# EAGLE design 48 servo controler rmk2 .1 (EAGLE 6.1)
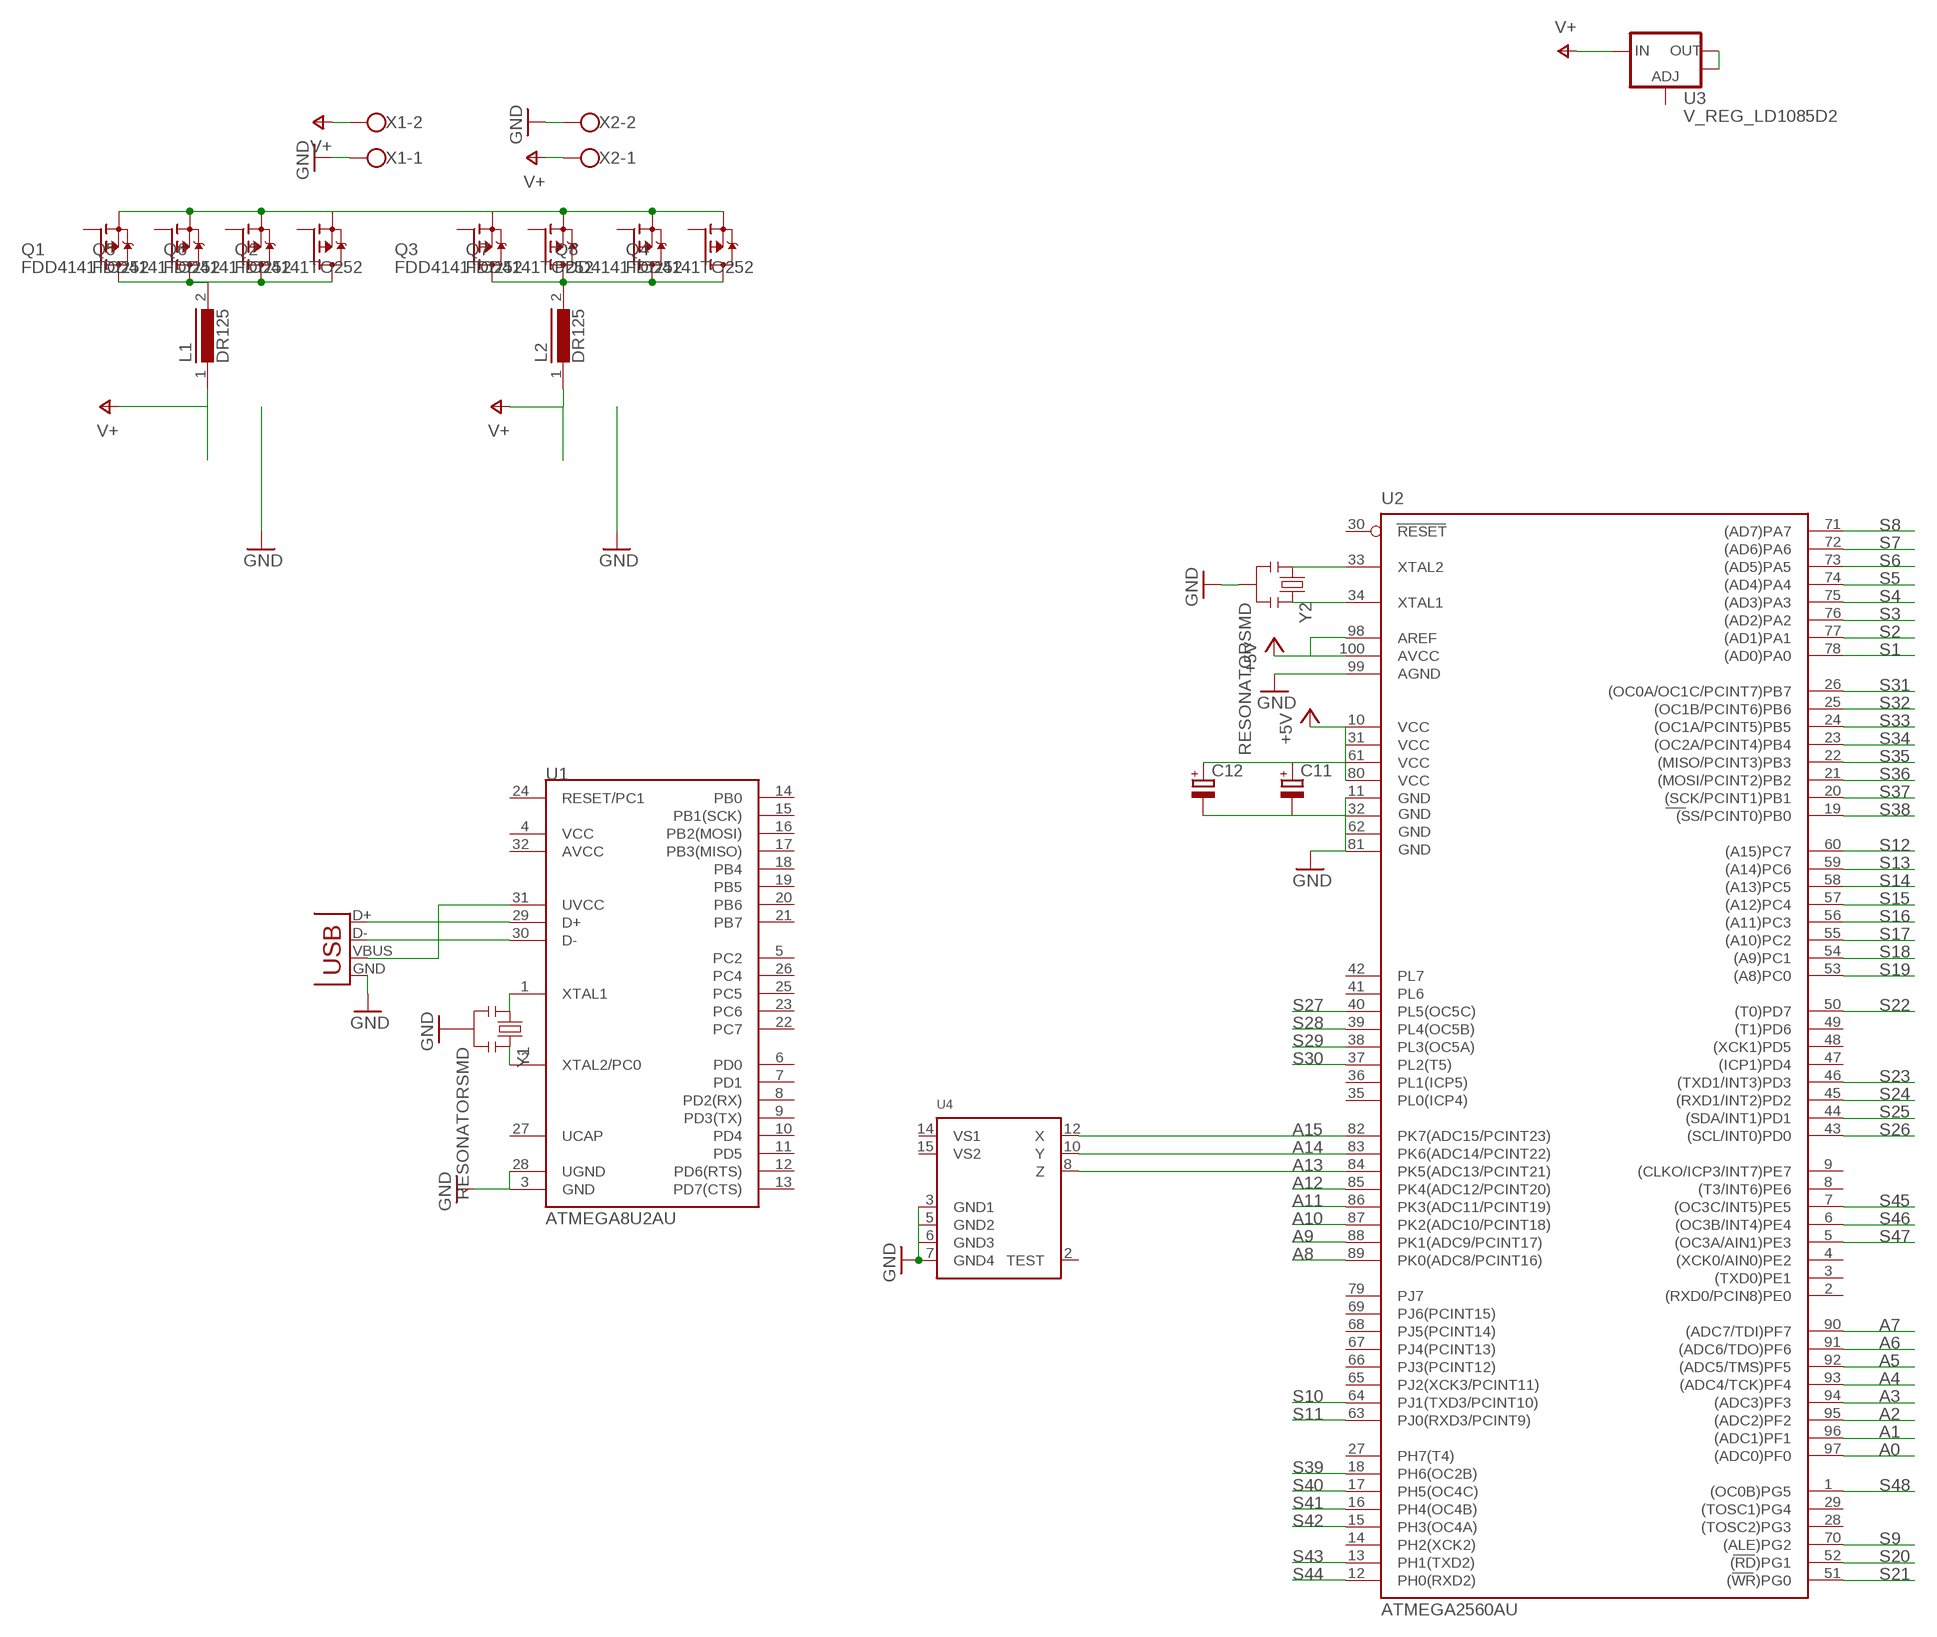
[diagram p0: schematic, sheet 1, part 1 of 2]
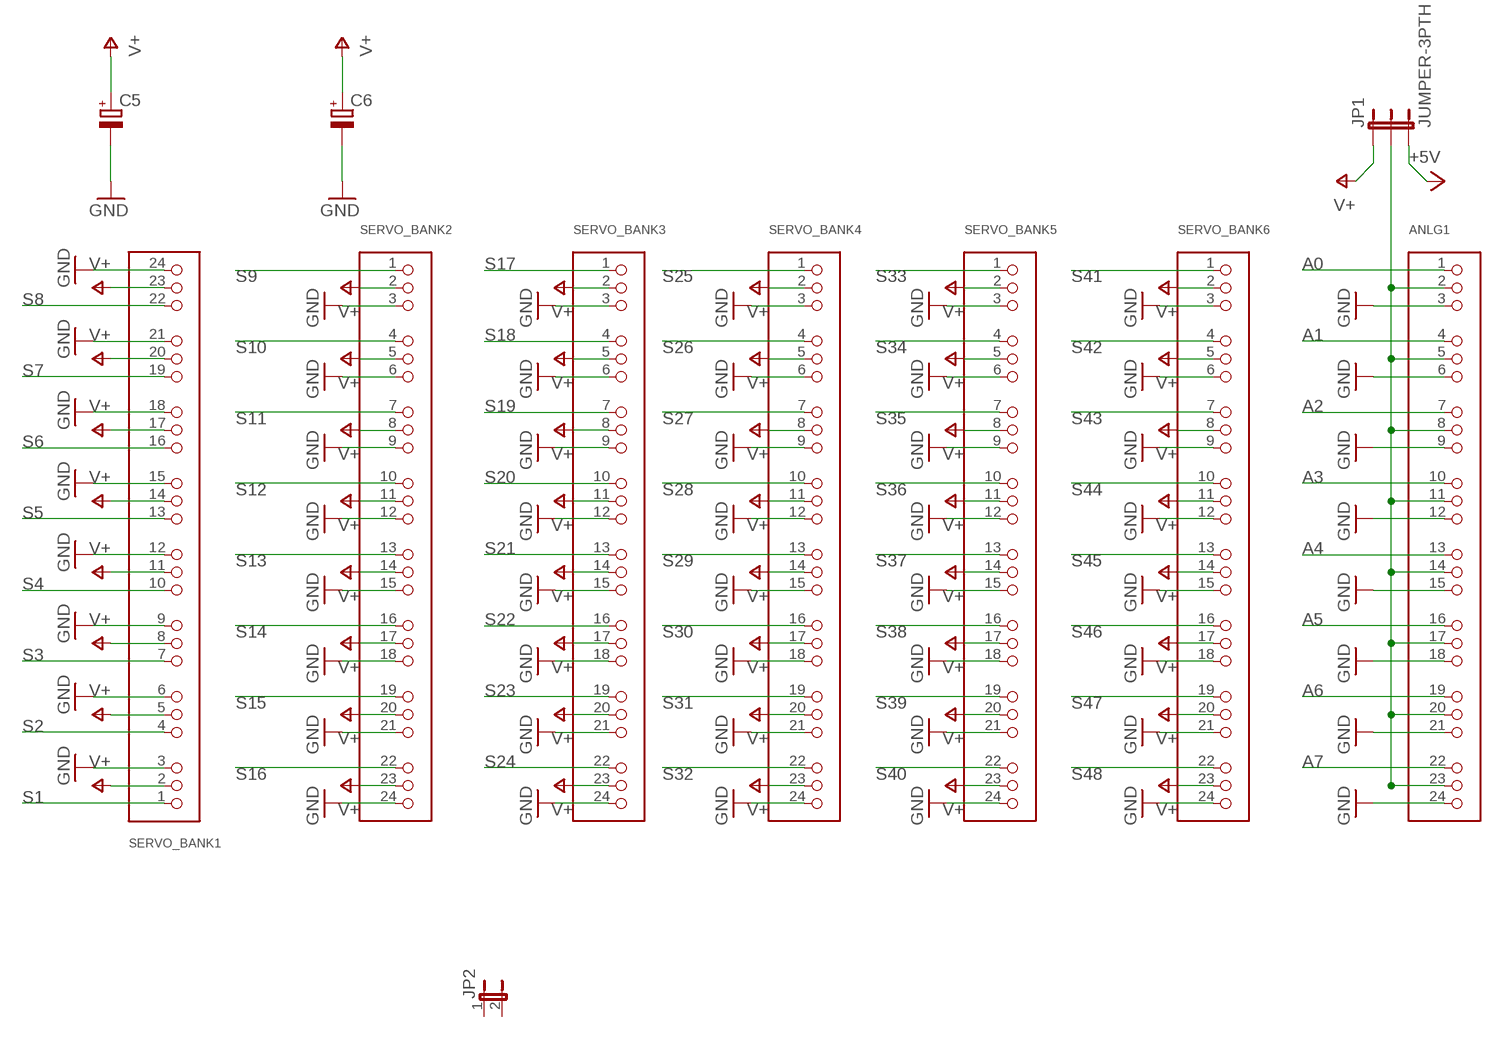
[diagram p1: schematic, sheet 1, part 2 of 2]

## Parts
ANLG1  HEADER-3X08  [3X08]
C5  CPOL-EUE5-8.5  [E5-8,5]
C6  CPOL-EUE5-8.5  [E5-8,5]
C11  CPOL-EUSMCE  [SMC_E]
C12  CPOL-EUSMCE  [SMC_E]
JP1  JUMPER-3PTH  [1X03]
JP2  JP1E  [JP1]
L1  DR125  [DR125]
L2  DR125  [DR125]
Q1  FDD4141TO252  [TO252]
Q2  FDD4141TO252  [TO252]
Q3  FDD4141TO252  [TO252]
Q4  FDD4141TO252  [TO252]
Q5  FDD4141TO252  [TO252]
Q6  FDD4141TO252  [TO252]
Q7  FDD4141TO252  [TO252]
Q8  FDD4141TO252  [TO252]
SERVO_BANK1  HEADER-3X08  [3X08]
SERVO_BANK2  HEADER-3X08  [3X08]
SERVO_BANK3  HEADER-3X08  [3X08]
SERVO_BANK4  HEADER-3X08  [3X08]
SERVO_BANK5  HEADER-3X08  [3X08]
SERVO_BANK6  HEADER-3X08  [3X08]
U1  ATMEGA8U2AU  [TQFP32-08]
U2  ATMEGA2560AU  [TQFP100]
U3  V_REG_LD1085D2  [D2PACK/A]
U4  ACCEL_ADXL335WAVE  [LFCSP16-W]
X1  W237-102  [W237-102]
X2  W237-102  [W237-102]
X4  USBSMD  [USB-MINIB]
Y1  RESONATORSMD  [RESONATOR-SMD]
Y2  RESONATORSMD  [RESONATOR-SMD]

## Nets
+5V: C11.+ C12.+ JP1.3 U2.10(VCC) U2.31(VCC1) U2.61(VCC2) U2.80(VCC3) U2.98(AREF) U2.100(AVCC)
A0: ANLG1.1 U2.97((ADC0)PF0)
A1: ANLG1.4 U2.96((ADC1)PF1)
A2: ANLG1.7 U2.95((ADC2)PF2)
A3: ANLG1.10 U2.94((ADC3)PF3)
A4: ANLG1.13 U2.93((ADC4/TCK)PF4)
A5: ANLG1.16 U2.92((ADC5/TMS)PF5)
A6: ANLG1.19 U2.91((ADC6/TDO)PF6)
A7: ANLG1.22 U2.90((ADC7/TDI)PF7)
A8: U2.89(PK0(ADC8/PCINT16))
A9: U2.88(PK1(ADC9/PCINT17))
A10: U2.87(PK2(ADC10/PCINT18))
A11: U2.86(PK3(ADC11/PCINT19))
A12: U2.85(PK4(ADC12/PCINT20))
A13: U2.84(PK5(ADC13/PCINT21)) U4.8(Z)
A14: U2.83(PK6(ADC14/PCINT22)) U4.10(Y)
A15: U2.82(PK7(ADC15/PCINT23)) U4.12(X)
GND: ANLG1.3 ANLG1.6 ANLG1.9 ANLG1.12 ANLG1.15 ANLG1.18 ANLG1.21 ANLG1.24 C5.- C6.- C11.- C12.- SERVO_BANK1.3 SERVO_BANK1.6 SERVO_BANK1.9 SERVO_BANK1.12 SERVO_BANK1.15 SERVO_BANK1.18 SERVO_BANK1.21 SERVO_BANK1.24 SERVO_BANK2.3 SERVO_BANK2.6 SERVO_BANK2.9 SERVO_BANK2.12 SERVO_BANK2.15 SERVO_BANK2.18 SERVO_BANK2.21 SERVO_BANK2.24 SERVO_BANK3.3 SERVO_BANK3.6 SERVO_BANK3.9 SERVO_BANK3.12 SERVO_BANK3.15 SERVO_BANK3.18 SERVO_BANK3.21 SERVO_BANK3.24 SERVO_BANK4.3 SERVO_BANK4.6 SERVO_BANK4.9 SERVO_BANK4.12 SERVO_BANK4.15 SERVO_BANK4.18 SERVO_BANK4.21 SERVO_BANK4.24 SERVO_BANK5.3 SERVO_BANK5.6 SERVO_BANK5.9 SERVO_BANK5.12 SERVO_BANK5.15 SERVO_BANK5.18 SERVO_BANK5.21 SERVO_BANK5.24 SERVO_BANK6.3 SERVO_BANK6.6 SERVO_BANK6.9 SERVO_BANK6.12 SERVO_BANK6.15 SERVO_BANK6.18 SERVO_BANK6.21 SERVO_BANK6.24 U1.3(GND) U1.28(UGND) U2.11(GND) U2.32(GND1) U2.62(GND2) U2.81(GND3) U2.99(AGND) U4.3(GND1) U4.5(GND2) U4.6(GND3) U4.7(GND4) X1.1 X2.2 X4.GND Y1.2 Y2.2
N$1: U2.34(XTAL1) Y2.3
N$2: U2.33(XTAL2) Y2.1
N$3: U1.2(XTAL2/PC0) Y1.3
N$4: U1.1(XTAL1) Y1.1
N$5: U3.2(OUT) U3.TAB(OUT)
N$9: U1.29(D+) X4.D+
N$10: ANLG1.2 ANLG1.5 ANLG1.8 ANLG1.11 ANLG1.14 ANLG1.17 ANLG1.20 ANLG1.23 JP1.2
N$11: U1.30(D-) X4.D-
N$12: U1.31(UVCC) X4.VBUS
N$49: L2.2 Q3.3(D) Q4.3(D) Q7.3(D) Q8.3(D)
N$50: L1.2 Q1.3(D) Q2.3(D) Q5.3(D) Q6.3(D)
N$51: Q1.2(S) Q2.2(S) Q3.2(S) Q4.2(S) Q5.2(S) Q6.2(S) Q7.2(S) Q8.2(S)
S1: SERVO_BANK1.1 U2.78((AD0)PA0)
S2: SERVO_BANK1.4 U2.77((AD1)PA1)
S3: SERVO_BANK1.7 U2.76((AD2)PA2)
S4: SERVO_BANK1.10 U2.75((AD3)PA3)
S5: SERVO_BANK1.13 U2.74((AD4)PA4)
S6: SERVO_BANK1.16 U2.73((AD5)PA5)
S7: SERVO_BANK1.19 U2.72((AD6)PA6)
S8: SERVO_BANK1.22 U2.71((AD7)PA7)
S9: SERVO_BANK2.1 U2.70((ALE)PG2)
S10: SERVO_BANK2.4 U2.64(PJ1(TXD3/PCINT10))
S11: SERVO_BANK2.7 U2.63(PJ0(RXD3/PCINT9))
S12: SERVO_BANK2.10 U2.60((A15)PC7)
S13: SERVO_BANK2.13 U2.59((A14)PC6)
S14: SERVO_BANK2.16 U2.58((A13)PC5)
S15: SERVO_BANK2.19 U2.57((A12)PC4)
S16: SERVO_BANK2.22 U2.56((A11)PC3)
S17: SERVO_BANK3.1 U2.55((A10)PC2)
S18: SERVO_BANK3.4 U2.54((A9)PC1)
S19: SERVO_BANK3.7 U2.53((A8)PC0)
S20: SERVO_BANK3.10 U2.52((RD)PG1)
S21: SERVO_BANK3.13 U2.51((WR)PG0)
S22: SERVO_BANK3.16 U2.50((T0)PD7)
S23: SERVO_BANK3.19 U2.46((TXD1/INT3)PD3)
S24: SERVO_BANK3.22 U2.45((RXD1/INT2)PD2)
S25: SERVO_BANK4.1 U2.44((SDA/INT1)PD1)
S26: SERVO_BANK4.4 U2.43((SCL/INT0)PD0)
S27: SERVO_BANK4.7 U2.40(PL5(OC5C))
S28: SERVO_BANK4.10 U2.39(PL4(OC5B))
S29: SERVO_BANK4.13 U2.38(PL3(OC5A))
S30: SERVO_BANK4.16 U2.37(PL2(T5))
S31: SERVO_BANK4.19 U2.26((OC0A/OC1C/PCINT7)PB7)
S32: SERVO_BANK4.22 U2.25((OC1B/PCINT6)PB6)
S33: SERVO_BANK5.1 U2.24((OC1A/PCINT5)PB5)
S34: SERVO_BANK5.4 U2.23((OC2A/PCINT4)PB4)
S35: SERVO_BANK5.7 U2.22((MISO/PCINT3)PB3)
S36: SERVO_BANK5.10 U2.21((MOSI/PCINT2)PB2)
S37: SERVO_BANK5.13 U2.20((SCK/PCINT1)PB1)
S38: SERVO_BANK5.16 U2.19((SS/PCINT0)PB0)
S39: SERVO_BANK5.19 U2.18(PH6(OC2B))
S40: SERVO_BANK5.22 U2.17(PH5(OC4C))
S41: SERVO_BANK6.1 U2.16(PH4(OC4B))
S42: SERVO_BANK6.4 U2.15(PH3(OC4A))
S43: SERVO_BANK6.7 U2.13(PH1(TXD2))
S44: SERVO_BANK6.10 U2.12(PH0(RXD2))
S45: SERVO_BANK6.13 U2.7((OC3C/INT5)PE5)
S46: SERVO_BANK6.16 U2.6((OC3B/INT4)PE4)
S47: SERVO_BANK6.19 U2.5((OC3A/AIN1)PE3)
S48: SERVO_BANK6.22 U2.1((OC0B)PG5)
V+: C5.+ C6.+ JP1.1 L1.1 L2.1 SERVO_BANK1.2 SERVO_BANK1.5 SERVO_BANK1.8 SERVO_BANK1.11 SERVO_BANK1.14 SERVO_BANK1.17 SERVO_BANK1.20 SERVO_BANK1.23 SERVO_BANK2.2 SERVO_BANK2.5 SERVO_BANK2.8 SERVO_BANK2.11 SERVO_BANK2.14 SERVO_BANK2.17 SERVO_BANK2.20 SERVO_BANK2.23 SERVO_BANK3.2 SERVO_BANK3.5 SERVO_BANK3.8 SERVO_BANK3.11 SERVO_BANK3.14 SERVO_BANK3.17 SERVO_BANK3.20 SERVO_BANK3.23 SERVO_BANK4.2 SERVO_BANK4.5 SERVO_BANK4.8 SERVO_BANK4.11 SERVO_BANK4.14 SERVO_BANK4.17 SERVO_BANK4.20 SERVO_BANK4.23 SERVO_BANK5.2 SERVO_BANK5.5 SERVO_BANK5.8 SERVO_BANK5.11 SERVO_BANK5.14 SERVO_BANK5.17 SERVO_BANK5.20 SERVO_BANK5.23 SERVO_BANK6.2 SERVO_BANK6.5 SERVO_BANK6.8 SERVO_BANK6.11 SERVO_BANK6.14 SERVO_BANK6.17 SERVO_BANK6.20 SERVO_BANK6.23 U3.3(IN) X1.2 X2.1
Unconnected: JP2.1 JP2.2 Q1.1(G) Q2.1(G) Q3.1(G) Q4.1(G) Q5.1(G) Q6.1(G) Q7.1(G) Q8.1(G) U1.4(VCC) U1.5(PC2) U1.6(PD0) U1.7(PD1) U1.8(PD2(RX)) U1.9(PD3(TX)) U1.10(PD4) U1.11(PD5) U1.12(PD6(RTS)) U1.13(PD7(CTS)) U1.14(PB0) U1.15(PB1(SCK)) U1.16(PB2(MOSI)) U1.17(PB3(MISO)) U1.18(PB4) U1.19(PB5) U1.20(PB6) U1.21(PB7) U1.22(PC7) U1.23(PC6) U1.24(RESET/PC1) U1.25(PC5) U1.26(PC4) U1.27(UCAP) U1.32(AVCC) U2.2((RXD0/PCIN8)PE0) U2.3((TXD0)PE1) U2.4((XCK0/AIN0)PE2) U2.8((T3/INT6)PE6) U2.9((CLKO/ICP3/INT7)PE7) U2.14(PH2(XCK2)) U2.27(PH7(T4)) U2.28((TOSC2)PG3) U2.29((TOSC1)PG4) U2.30(RESET) U2.35(PL0(ICP4)) U2.36(PL1(ICP5)) U2.41(PL6) U2.42(PL7) U2.47((ICP1)PD4) U2.48((XCK1)PD5) U2.49((T1)PD6) U2.65(PJ2(XCK3/PCINT11)) U2.66(PJ3(PCINT12)) U2.67(PJ4(PCINT13)) U2.68(PJ5(PCINT14)) U2.69(PJ6(PCINT15)) U2.79(PJ7) U3.1(ADJ) U4.2(TEST) U4.14(VS1) U4.15(VS2)

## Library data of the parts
ANLG1 SERVO_BANK1-SERVO_BANK6 = microbuilder:HEADER-3X08: 3x8 0.1" Headers Male - 4UCON: 01058
C5 C6 C11 C12 = resistor:CPOL-EU: POLARIZED CAPACITOR, European symbol
JP1 = SparkFun:JUMPER-3
JP2 = jumper:JP1E: JUMPER
L1 L2 = inductors:DR125: High Power Density, High Efficiency, Shielded Inductors
Q1-Q8 = transistor-fet:FDD4141: P-Channel PowerTrench® MOSFET Source: FDD4141.pdf
U1 = SparkFun:ATMEGA8U2: Atmel 8-bit Microcontroller with 8/16/32K Bystes of ISP Flash and USB Controller. ATmega8U2, ATmega16U2, and ATmega32U2
U2 = SparkFun:ATMEGA2560: MICROCONTROLLER 64/128/256 Kbytes FLASH 4 Kbytes EEPROM 8 Kbytes SRAM 86 General Purpose I/O pins 12-channels16-bit PWM 4 x Serial USARTs 16-channels 10-bit A/D
U3 = SparkFun:V_REG_LD1085: LD1085 3A low-drop positive voltage regulator, adjustable The LD1085xx is a low drop voltage regulator able to provide up to 3 A of output current. Dropout is guaranteed at a maximum of 1.2 V at the maximum output current, decreasing at lower loads. The LD1085xx is pin to pin compatible with the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
U4 = microbuilder:ACCEL_ADXL335: ADXL335 Low-Power 3 Axis Accelerometer LFCSP16-R - 16 Pin LFCSP Package (Reflow footprint) LFSCP16-W - 16 Pin LFCSP Package (Wave footprint with extended pads for hand soldering) Digikey: ADXL335BCPZ-RL7CT-ND
X1 X2 = con-wago-500:W237-102: WAGO SCREW CLAMP; MPN: 237-102; OC_FARNELL: unknown; OC_NEWARK: 70K9898
X4 = SparkFun:USB: USB Connectors USB-B-PTH is fully proven SKU : PRT-00139 USB-miniB is fully proven SKU : PRT-00587 USB-A-PCB is untested. USB-A-H is throughly reviewed, but untested. Spark Fun Electronics SKU : PRT-00437 USB-B-SMT is throughly reviewed, but untested. Needs silkscreen touching up. USB-A-S has not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
Y1 Y2 = SparkFun:RESONATOR: Resonator Small SMD resonator. This is the itty bitty 10/20MHz resonators with built in caps. CSTCE10M0G55 and CSTCE20M0V53. Footprint has been reviewed closely but hasn't been tested yet.

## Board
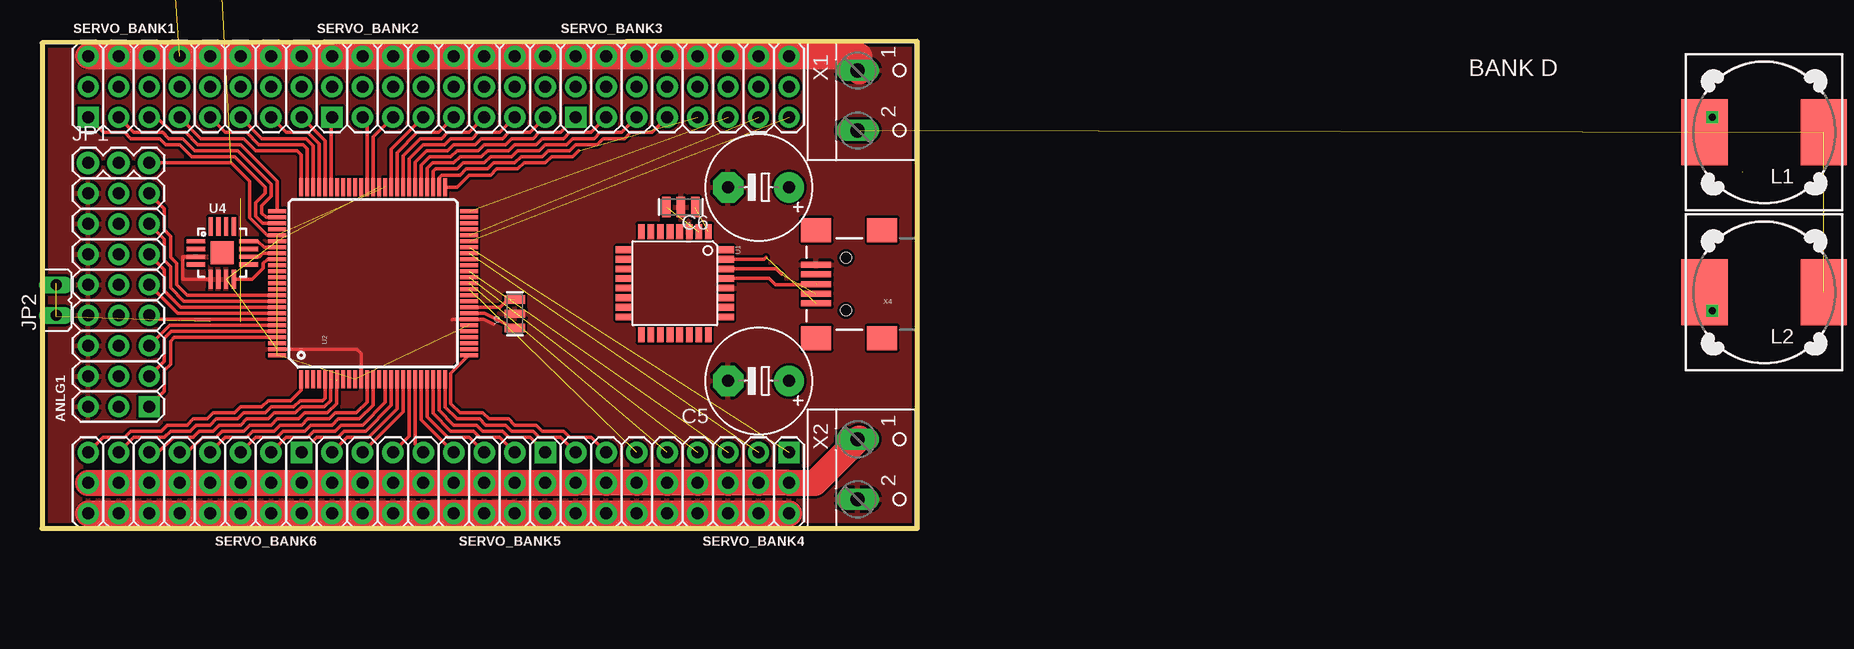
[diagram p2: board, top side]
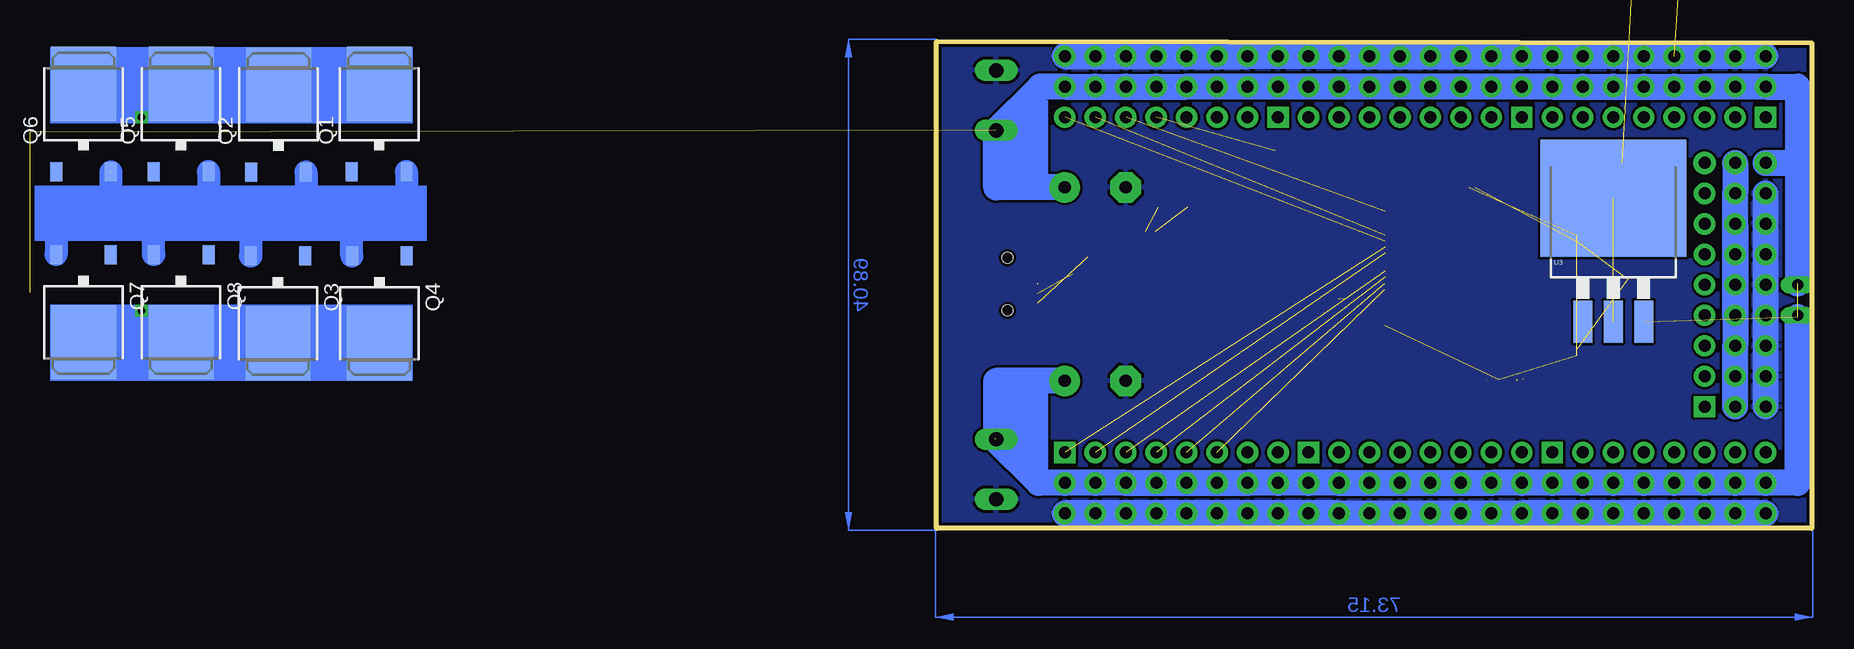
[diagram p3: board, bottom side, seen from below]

Size 72.95 x 40.57 mm. Coordinates in mm from the lower left corner, seen from the top.
Outline: 0,40.44 0,0 72.95,0 72.95,40.57 0,40.44
Copper layers (1*16): Top 0.035mm / dielectric 1.5mm / Bottom 0.035mm
Design rules: minimum track width 10mil, minimum drill 24mil, track to track 8mil, track to pad 8mil, pad to pad 8mil, via to via 8mil, smd to smd 8mil, copper to edge 10mil, drill to drill 8mil, minimum pad ring 10mil, minimum via ring 8mil, stop-mask expansion 4mil, vias tented up to drill 0mil, thermal gap 10mil

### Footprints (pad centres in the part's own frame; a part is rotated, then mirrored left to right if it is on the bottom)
3X08 = drill 1 pad 1.778 square: 1 -8.89,-2.54 | drill 1 pad 1.778: 2 -8.89,0; 3 -8.89,2.54; 4 -6.35,-2.54; 5 -6.35,0; 6 -6.35,2.54; 7 -3.81,-2.54; 8 -3.81,0; 9 -3.81,2.54; 10 -1.27,-2.54; 11 -1.27,0; 12 -1.27,2.54; 13 1.27,-2.54; 14 1.27,0; 15 1.27,2.54; 16 3.81,-2.54; 17 3.81,0; 18 3.81,2.54; 19 6.35,-2.54; 20 6.35,0; 21 6.35,2.54; 22 8.89,-2.54; 23 8.89,0; 24 8.89,2.54
E5-8,5 = drill 1.016 pad 2.54: + -2.54,0 | drill 1.016 pad 2.54 octagon: - 2.54,0
SMC_E = smd 2.4 x 2.8: + -3.15,0; - 3.15,0
1X03 = drill 1.016 pad 1.88: 1 0,0; 2 2.54,0; 3 5.08,0
JP1 = drill 0.914 long: 1 0,-1.27; 2 0,1.27
DR125 = smd 3.85 x 5.5: 1 -4.975,0; 2 4.975,0
TO252 = smd 1 x 1.6: 1 -2.28,-4.8; 2 2.28,-4.8 | smd 5.4 x 6.2: 3 0,2.5
TQFP32-08 = smd 1.27 x 0.559: 1 -4.293,2.8; 2 -4.293,2; 3 -4.293,1.2; 4 -4.293,0.4; 5 -4.293,-0.4; 6 -4.293,-1.2; 7 -4.293,-2; 8 -4.293,-2.8; 17 4.293,-2.8; 18 4.293,-2; 19 4.293,-1.2; 20 4.293,-0.4; 21 4.293,0.4; 22 4.293,1.2; 23 4.293,2; 24 4.293,2.8 | smd 0.559 x 1.27: 9 -2.8,-4.293; 10 -2,-4.293; 11 -1.2,-4.293; 12 -0.4,-4.293; 13 0.4,-4.293; 14 1.2,-4.293; 15 2,-4.293; 16 2.8,-4.293; 25 2.8,4.293; 26 2,4.293; 27 1.2,4.293; 28 0.4,4.293; 29 -0.4,4.293; 30 -1.2,4.293; 31 -2,4.293; 32 -2.8,4.293
TQFP100 = smd 1.5 x 0.3: 1 -8,6; 2 -8,5.5; 3 -8,5; 4 -8,4.5; 5 -8,4; 6 -8,3.5; 7 -8,3; 8 -8,2.5; 9 -8,2; 10 -8,1.5; 11 -8,1; 12 -8,0.5; 13 -8,0; 14 -8,-0.5; 15 -8,-1; 16 -8,-1.5; 17 -8,-2; 18 -8,-2.5; 19 -8,-3; 20 -8,-3.5; 21 -8,-4; 22 -8,-4.5; 23 -8,-5; 24 -8,-5.5; 25 -8,-6; 51 8,-6; 52 8,-5.5; 53 8,-5; 54 8,-4.5; 55 8,-4; 56 8,-3.5; 57 8,-3; 58 8,-2.5; 59 8,-2; 60 8,-1.5; 61 8,-1; 62 8,-0.5; 63 8,0; 64 8,0.5; 65 8,1; 66 8,1.5; 67 8,2; 68 8,2.5; 69 8,3; 70 8,3.5; 71 8,4; 72 8,4.5; 73 8,5; 74 8,5.5; 75 8,6 | smd 0.3 x 1.5: 26 -6,-8; 27 -5.5,-8; 28 -5,-8; 29 -4.5,-8; 30 -4,-8; 31 -3.5,-8; 32 -3,-8; 33 -2.5,-8; 34 -2,-8; 35 -1.5,-8; 36 -1,-8; 37 -0.5,-8; 38 0,-8; 39 0.5,-8; 40 1,-8; 41 1.5,-8; 42 2,-8; 43 2.5,-8; 44 3,-8; 45 3.5,-8; 46 4,-8; 47 4.5,-8; 48 5,-8; 49 5.5,-8; 50 6,-8; 76 6,8; 77 5.5,8; 78 5,8; 79 4.5,8; 80 4,8; 81 3.5,8; 82 3,8; 83 2.5,8; 84 2,8; 85 1.5,8; 86 1,8; 87 0.5,8; 88 0,8; 89 -0.5,8; 90 -1,8; 91 -1.5,8; 92 -2,8; 93 -2.5,8; 94 -3,8; 95 -3.5,8; 96 -4,8; 97 -4.5,8; 98 -5,8; 99 -5.5,8; 100 -6,8
D2PACK/A = smd 1.6 x 3.5: 1 -2.54,-8.275; 2 0,-8.275; 3 2.54,-8.275 | smd 12.2 x 9.75: TAB 0,2
LFCSP16-W = smd 1.9 x 1.9: 0 0,0 | smd 1.558 x 0.35: 1 -2.204,0.975; 2 -2.204,0.325; 3 -2.204,-0.325; 4 -2.204,-0.975; 9 2.204,-0.975; 10 2.204,-0.325; 11 2.204,0.325; 12 2.204,0.975 | smd 0.35 x 1.558: 5 -0.975,-2.204; 6 -0.325,-2.204; 7 0.325,-2.204; 8 0.975,-2.204; 13 0.975,2.204; 14 0.325,2.204; 15 -0.325,2.204; 16 -0.975,2.204
W237-102 = drill 1.194 long: 1 -2.5,-1.27; 2 2.5,-1.27
USB-MINIB = smd 2.5 x 0.5: D+ 2.5,0; D- 2.5,0.8; GND 2.5,-1.6; ID 2.5,-0.8; VBUS 2.5,1.6 | smd 2.5 x 2: MTN1 -3,4.5; MTN2 2.5,4.5; MTN3 -3,-4.5; MTN4 2.5,-4.5 | hole 0.9: 0,2.2; 0,-2.2
RESONATOR-SMD = smd 0.7 x 1.7: 1 -1.2,0; 2 0,0; 3 1.2,0

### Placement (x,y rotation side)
ANLG1  6.38,19.02 90 top
C5  59.72,12.29 180 top
C6  59.72,28.42 180 top
C11  not placed on the board
C12  not placed on the board
JP1  3.84,30.45 0 top
JP2  1.17,19.02 0 top
L1  143.54,32.99 180 top  (outside the outline)
L2  143.54,19.65 180 top  (outside the outline)
Q1  119.41,34.51 0 bottom  (outside the outline)
Q2  127.79,34.48 0 bottom  (outside the outline)
Q3  127.85,17.91 180 bottom  (outside the outline)
Q4  119.4,17.91 180 bottom  (outside the outline)
Q5  135.92,34.51 0 bottom  (outside the outline)
Q6  144.05,34.51 0 bottom  (outside the outline)
Q7  144.05,18 180 bottom  (outside the outline)
Q8  135.92,18 180 bottom  (outside the outline)
SERVO_BANK1  12.73,36.8 0 top
SERVO_BANK2  33.05,36.8 0 top
SERVO_BANK3  53.37,36.8 0 top
SERVO_BANK4  53.37,3.78 180 top
SERVO_BANK5  33.05,3.78 180 top
SERVO_BANK6  12.73,3.78 180 top
U1  52.73,20.41 270 top
U2  27.59,20.41 90 top
U3  16.54,25.49 0 bottom
U4  15.01,22.95 0 top
X1  69.24,35.65 270 top
X2  69.24,4.92 270 top
X4  67.02,20.35 180 top
Y1  53.24,26.76 180 top
Y2  39.4,17.87 90 top

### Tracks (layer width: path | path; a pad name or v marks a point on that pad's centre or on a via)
+5V  (7 unrouted)
  Top 0.305: U2.80 18.76,24.41 17.3,25.88 17.3,28.92 15.78,30.45 JP1.3
A0
  Top 0.305: U2.97 11.02,15.91 10.7,15.59 10.7,13.68 10.19,13.17 10.19,11.4 ANLG1.1
A1
  Top 0.305: U2.96 10.76,16.41 10.19,15.84 10.19,13.94 ANLG1.4
A2
  Top 0.305: U2.95 10.62,16.91 ANLG1.7
A3
  Top 0.305: U2.94 9.25,17.41 ANLG1.10
A4
  Top 0.305: U2.93 11.29,17.91 ANLG1.13
A5
  Top 0.305: U2.92 11.55,18.41 10.19,19.78 10.19,21.56 ANLG1.16
A6
  Top 0.305: U2.91 11.81,18.91 10.7,20.03 10.7,21.81 10.19,22.32 10.19,24.1 ANLG1.19
A7
  Top 0.305: U2.90 12.08,19.41 11.2,20.29 11.2,22.07 10.7,22.57 10.7,24.35 10.19,24.86 10.19,26.64 ANLG1.22
A13
  Top 0.305: U4.8 17.51,20.75 18.44,21.68 18.44,22.07 18.79,22.41 U2.84
A14
  Top 0.305: U4.10 18.12,22.63 18.4,22.91 U2.83
A15
  Top 0.305: U2.82 18.49,23.41 17.98,23.93 U4.12
GND  (5 unrouted)
  Top 0.305: 37.62,16.98 36.81,17.41 U2.32 34.24,17.41 34.19,17.37 | U2.99 26.23,14.91 26.57,14.57 26.57,12.43 U2.11 | U4.3 11.71,22.63 11.71,20.75 U4.5
  Top 2.184: SERVO_BANK6.24 SERVO_BANK6.21 SERVO_BANK6.18 SERVO_BANK6.15 SERVO_BANK6.12 SERVO_BANK6.9 SERVO_BANK6.6 SERVO_BANK6.3 SERVO_BANK5.24 SERVO_BANK5.21 SERVO_BANK5.18 SERVO_BANK5.15 SERVO_BANK5.12 SERVO_BANK5.9 SERVO_BANK5.6 SERVO_BANK5.3 SERVO_BANK4.24 SERVO_BANK4.21 SERVO_BANK4.18 SERVO_BANK4.15 SERVO_BANK4.12 SERVO_BANK4.9 SERVO_BANK4.6 SERVO_BANK4.3 | SERVO_BANK1.3 SERVO_BANK1.6 SERVO_BANK1.9 SERVO_BANK1.12 SERVO_BANK1.15 SERVO_BANK1.18 SERVO_BANK1.21 SERVO_BANK1.24 SERVO_BANK2.3 SERVO_BANK2.6 SERVO_BANK2.9 SERVO_BANK2.12 SERVO_BANK2.15 SERVO_BANK2.18 SERVO_BANK2.21 SERVO_BANK2.24 SERVO_BANK3.3 SERVO_BANK3.6 SERVO_BANK3.9 SERVO_BANK3.12 SERVO_BANK3.15 SERVO_BANK3.18 SERVO_BANK3.21 SERVO_BANK3.24 68.1,39.34 68.1,38.07
  Bottom 2.184: SERVO_BANK1.3 SERVO_BANK1.6 SERVO_BANK1.9 SERVO_BANK1.12 SERVO_BANK1.15 SERVO_BANK1.18 SERVO_BANK1.21 SERVO_BANK1.24 SERVO_BANK2.3 SERVO_BANK2.6 SERVO_BANK2.9 SERVO_BANK2.12 SERVO_BANK2.15 SERVO_BANK2.18 SERVO_BANK2.21 SERVO_BANK2.24 SERVO_BANK3.3 SERVO_BANK3.6 SERVO_BANK3.9 SERVO_BANK3.12 SERVO_BANK3.15 SERVO_BANK3.18 SERVO_BANK3.21 SERVO_BANK3.24 | SERVO_BANK4.24 SERVO_BANK4.21 SERVO_BANK4.18 SERVO_BANK4.15 | SERVO_BANK4.15 SERVO_BANK4.12 SERVO_BANK4.9 SERVO_BANK4.6 SERVO_BANK4.3 | SERVO_BANK4.24 SERVO_BANK4.15 | SERVO_BANK6.24 SERVO_BANK6.21 SERVO_BANK6.18 SERVO_BANK6.15 SERVO_BANK6.12 SERVO_BANK6.9 SERVO_BANK6.6 SERVO_BANK6.3 SERVO_BANK5.24 SERVO_BANK5.21 SERVO_BANK5.18 SERVO_BANK5.15 SERVO_BANK5.12 SERVO_BANK5.9 SERVO_BANK5.6 SERVO_BANK5.3 SERVO_BANK4.24 | ANLG1.3 ANLG1.6 ANLG1.9 ANLG1.12 ANLG1.15 ANLG1.18 ANLG1.21 ANLG1.24
  pour Top: -0.1,40.48 73.05,40.73 73.05,-0.16 -0.1,-0.16
  pour Bottom: 0.15,40.35 72.93,40.35 72.93,0.09 0.28,0.09 0.28,40.23
N$1  (1 unrouted)
  Top 0.305: U2.34 38.16,18.41 38.89,19.14
N$2
  Top 0.305: U2.33 36.89,17.91 Y2.1
N$3  (1 unrouted)
N$4  (1 unrouted)
N$5  (1 unrouted)
N$9  (1 unrouted)
  Top 0.305: U1.29 60.59,20.81 61.12,20.29 64.42,20.29 64.54,20.41
N$10
  Bottom 2.184: ANLG1.20 ANLG1.17 ANLG1.14 ANLG1.11 | ANLG1.11 ANLG1.8 ANLG1.5 ANLG1.2 | ANLG1.11 ANLG1.23 JP1.2
N$11  (1 unrouted)
  Top 0.305: U1.30 61.19,21.61 61.62,21.18
N$12  (1 unrouted)
  Top 0.305: U1.31 60.19,22.41 60.35,22.57
N$49  (via drill 0.6)
  Top 0.254: L2.2 138.97,19.91 v139.22,18.13
  Bottom 0.254: Q8.3 139.22,15.5 v139.22,18.13
  Bottom 1.93: Q4.3 Q3.3 135.92,15.41 Q8.3 Q7.3
N$50  (via drill 0.6)
  Top 1.93: L1.2 138.46,34.26 v139.22,34.26
  Bottom 0.254: 135.92,36.98 139.22,36.98 v139.22,34.26
  Bottom 1.93: Q1.3 127.79,37.01 Q2.3 135.92,36.98 Q5.3 Q6.3
  Bottom 3.81: 135.92,37.05 Q5.3
N$51  (1 unrouted)
  Bottom 1.93: Q1.2 117.12,26.51 121.69,26.51 | 121.69,26.51 125.5,26.51 | 125.5,26.51 130.08,26.51 | 130.08,26.51 133.63,26.51 | 133.63,26.51 138.2,26.51 | 138.2,26.51 141.76,26.51 | 141.76,26.51 141.76,29.69 | Q2.2 125.5,26.51 | Q5.2 133.63,26.51 | Q4.2 121.69,22.71 121.69,26.51 | Q3.2 130.08,22.71 130.08,26.51 | Q8.2 138.2,26.51 | 141.76,26.51 146.33,26.51 Q7.2
S1
  Top 0.305: U2.78 18.4,25.41 17.81,26 17.81,27.14 18.57,27.91 18.57,28.42 16.03,30.96 12.47,30.96 11.46,31.97 10.31,31.97 9.81,32.48 7.39,32.48 6.89,32.99 5.11,32.99 SERVO_BANK1.1
S2
  Top 0.305: U2.77 18.66,25.91 18.32,26.26 18.32,26.89 19.08,27.65 19.08,28.67 16.28,31.46 12.73,31.46 11.71,32.48 10.57,32.48 10.06,32.99 7.65,32.99 SERVO_BANK1.4
S3
  Top 0.305: U2.76 19.59,28.92 16.54,31.97 12.98,31.97 11.97,32.99 10.82,32.99 9.55,34.26 SERVO_BANK1.7
S4
  Top 0.305: U2.75 21.59,31.11 21.24,31.46 17.81,31.46 16.79,32.48 13.24,32.48 SERVO_BANK1.10
S5
  Top 0.305: U2.74 22.09,31.63 21.75,31.97 18.06,31.97 17.05,32.99 15.27,32.99 SERVO_BANK1.13
S6
  Top 0.305: U2.73 22.59,31.89 22,32.48 18.32,32.48 SERVO_BANK1.16
S7
  Top 0.305: U2.72 23.09,32.03 22.13,32.99 20.35,32.99 SERVO_BANK1.19
S8
  Top 0.305: U2.71 23.59,32.29 SERVO_BANK1.22
S9
  Top 0.305: U2.70 24.09,34.19 SERVO_BANK2.1
S10
  Top 0.305: U2.64 27.09,33.87 SERVO_BANK2.4
S11
  Top 0.305: U2.63 27.59,32.61 SERVO_BANK2.7
S12
  Top 0.305: U2.60 29.09,31.57 SERVO_BANK2.10
S13
  Top 0.305: U2.59 29.59,31.3 31.27,32.99 33.05,32.99 SERVO_BANK2.13
S14
  Top 0.305: U2.58 30.09,31.04 31.52,32.48 33.3,32.48 33.81,32.99 35.59,32.99 SERVO_BANK2.16
S15
  Top 0.305: U2.57 30.59,30.78 31.78,31.97 33.56,31.97 34.06,32.48 35.84,32.48 36.35,32.99 38.13,32.99 SERVO_BANK2.19
S16
  Top 0.305: U2.56 31.09,30.52 32.03,31.46 33.81,31.46 34.32,31.97 36.1,31.97 36.6,32.48 38.38,32.48 38.89,32.99 40.67,32.99 SERVO_BANK2.22
S17
  Top 0.305: U2.55 31.59,30.26 32.29,30.96 34.06,30.96 34.57,31.46 36.35,31.46 36.86,31.97 38.64,31.97 39.14,32.48 40.92,32.48 41.43,32.99 43.21,32.99 SERVO_BANK3.1
S18
  Top 0.305: U2.54 32.09,29.99 32.54,30.45 34.32,30.45 34.83,30.96 36.6,30.96 37.11,31.46 38.89,31.46 39.4,31.97 41.18,31.97 41.68,32.48 43.46,32.48 43.97,32.99 45.75,32.99 SERVO_BANK3.4
S19
  Top 0.305: U2.53 32.59,29.73 32.79,29.94 34.57,29.94 35.08,30.45 36.86,30.45 37.37,30.96 39.14,30.96 39.65,31.46 41.43,31.46 41.94,31.97 43.72,31.97 44.22,32.48 46,32.48 46.51,32.99 48.29,32.99 SERVO_BANK3.7
S20
  Top 0.305: U2.52 33.09,29.22 33.3,29.43 34.83,29.43 35.33,29.94 37.11,29.94 37.62,30.45 39.4,30.45 39.91,30.96 41.68,30.96 42.19,31.46 43.97,31.46 44.48,31.97 46.26,31.97 46.76,32.48 48.54,32.48 49.05,32.99 50.83,32.99 SERVO_BANK3.10
S21  (1 unrouted)
  Top 0.305: U2.51 34.57,28.41 35.59,29.43 37.37,29.43 37.87,29.94 39.65,29.94 40.16,30.45 41.94,30.45 42.45,30.96 44.22,30.96 44.73,31.46
S22  (1 unrouted)
S23  (1 unrouted)
S24  (1 unrouted)
S25  (1 unrouted)
S26  (1 unrouted)
S27  (1 unrouted)
S28  (1 unrouted)
S29  (1 unrouted)
S30  (1 unrouted)
S31
  Top 0.305: U2.26 35.56,14.41 34.06,12.92 34.06,10.38 34.83,9.62 36.73,9.62 37.24,9.11 38.89,9.11 39.4,8.6 41.18,8.6 41.68,8.09 43.46,8.09 43.97,7.59 45.75,7.59 SERVO_BANK4.19
S32
  Top 0.305: U2.25 33.59,10.1 34.57,9.11 36.48,9.11 36.98,8.6 38.64,8.6 39.14,8.09 40.92,8.09 41.43,7.59 43.21,7.59 SERVO_BANK4.22
S33
  Top 0.305: U2.24 33.09,9.83 34.32,8.6 36.22,8.6 36.73,8.09 38.38,8.09 38.89,7.59 40.67,7.59 SERVO_BANK5.1
S34
  Top 0.305: SERVO_BANK5.4 38.13,7.59 36.48,7.59 35.97,8.09 34.06,8.09 32.59,9.57 U2.23
S35
  Top 0.305: U2.22 32.09,9.31 33.81,7.59 35.59,7.59 SERVO_BANK5.7
S36
  Top 0.305: U2.21 31.59,9.05 SERVO_BANK5.10
S37
  Top 0.305: U2.20 31.09,7.01 SERVO_BANK5.13
S38
  Top 0.305: U2.19 30.59,7.67 SERVO_BANK5.16
S39
  Top 0.305: U2.18 30.09,9.71 SERVO_BANK5.19
S40
  Top 0.305: U2.17 29.59,9.97 27.21,7.59 25.43,7.59 SERVO_BANK5.22
S41
  Top 0.305: U2.16 29.09,10.23 26.95,8.09 25.17,8.09 24.67,7.59 22.89,7.59 SERVO_BANK6.1
S42
  Top 0.305: U2.15 28.59,10.49 26.7,8.6 24.92,8.6 24.41,8.09 22.63,8.09 22.13,7.59 20.35,7.59 SERVO_BANK6.4
S43
  Top 0.305: U2.13 27.59,10.25 26.44,9.11 24.67,9.11 24.16,8.6 22.38,8.6 21.87,8.09 20.09,8.09 19.59,7.59 17.81,7.59 SERVO_BANK6.7
S44  (1 unrouted)
  Top 0.305: U2.12 27.08,10.51 26.19,9.62 24.41,9.62 23.9,9.11 22.13,9.11 21.62,8.6 19.84,8.6 19.33,8.09 17.55,8.09 17.05,7.59 15.27,7.59 SERVO_BANK6.10
S45  (1 unrouted)
  Top 0.305: 24.54,12.29 24.54,10.38 23.78,9.62 21.87,9.62 21.36,9.11 19.59,9.11 19.08,8.6 17.3,8.6 16.79,8.09 15.01,8.09 14.51,7.59 13.36,7.59 12.35,6.57 11.71,6.57 SERVO_BANK6.13
S46  (1 unrouted)
  Top 0.305: 24.03,12.41 24.03,10.63 23.52,10.13 21.62,10.13 21.11,9.62 19.33,9.62 18.82,9.11 17.05,9.11 16.54,8.6 14.76,8.6 14.25,8.09 13.11,8.09 12.6,7.59 10.95,7.59 9.68,6.32 SERVO_BANK6.16
S47
  Top 0.305: U2.5 23.59,10.83 23.4,10.63 21.49,10.63 20.98,10.13 19.08,10.13 18.57,9.62 16.79,9.62 16.28,9.11 14.51,9.11 14,8.6 12.85,8.6 12.35,8.09 10.7,8.09 10.19,7.59 7.65,7.59 SERVO_BANK6.19
S48
  Top 0.305: U2.1 21.59,11.49 20.73,10.63 18.82,10.63 18.32,10.13 16.54,10.13 16.03,9.62 14.25,9.62 13.74,9.11 12.6,9.11 12.09,8.6 10.44,8.6 9.93,8.09 7.39,8.09 6.89,7.59 5.11,7.59 SERVO_BANK6.22
V+  (5 unrouted)
  Top 2.184: SERVO_BANK6.23 SERVO_BANK6.20 SERVO_BANK6.17 SERVO_BANK6.14 SERVO_BANK6.11 SERVO_BANK6.8 SERVO_BANK6.5 SERVO_BANK6.2 SERVO_BANK5.23 SERVO_BANK5.20 SERVO_BANK5.17 SERVO_BANK5.14 SERVO_BANK5.11 SERVO_BANK5.8 SERVO_BANK5.5 SERVO_BANK5.2 SERVO_BANK4.23 SERVO_BANK4.20 SERVO_BANK4.17 SERVO_BANK4.14 SERVO_BANK4.11 SERVO_BANK4.8 SERVO_BANK4.5 SERVO_BANK4.2 64.42,3.78 68.1,7.46
  Bottom 2.184: 1.17,30.45 1.17,36.8 SERVO_BANK1.2 SERVO_BANK1.5 SERVO_BANK1.8 SERVO_BANK1.11 SERVO_BANK1.14 SERVO_BANK1.17 SERVO_BANK1.20 SERVO_BANK1.23 SERVO_BANK2.2 SERVO_BANK2.5 SERVO_BANK2.8 SERVO_BANK2.11 SERVO_BANK2.14 SERVO_BANK2.17 SERVO_BANK2.20 SERVO_BANK2.23 SERVO_BANK3.2 SERVO_BANK3.5 SERVO_BANK3.8 SERVO_BANK3.11 SERVO_BANK3.14 SERVO_BANK3.17 SERVO_BANK3.20 SERVO_BANK3.23 64.29,36.8 67.97,33.11 | JP1.1 1.17,30.45 | 1.17,17.62 1.17,3.78 SERVO_BANK6.23 SERVO_BANK6.20 SERVO_BANK6.17 SERVO_BANK6.14 SERVO_BANK6.11 SERVO_BANK6.8 SERVO_BANK6.5 SERVO_BANK6.2 SERVO_BANK5.23 SERVO_BANK5.20 SERVO_BANK5.17 SERVO_BANK5.14 SERVO_BANK5.11 SERVO_BANK5.8 SERVO_BANK5.5 SERVO_BANK5.2 SERVO_BANK4.23 SERVO_BANK4.20 SERVO_BANK4.17 SERVO_BANK4.14 SERVO_BANK4.11 SERVO_BANK4.8 SERVO_BANK4.5 SERVO_BANK4.2 64.42,3.78 68.1,7.46 | 1.17,30.45 1.17,20.41 | C6.+ 67.97,28.42 67.97,33.11 | X1.2 67.97,33.11 | C5.+ 67.97,12.29 X2.1
(copper drawn outside any net)
  shapes: Bottom area x7

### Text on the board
tNames: BANK D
